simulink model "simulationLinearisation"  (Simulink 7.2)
settings: Solver=ode23  StartTime=0.0  StopTime=2  RelTol=1e-3
undefined symbols (not defined in the file or in its folder): u_b, x_b

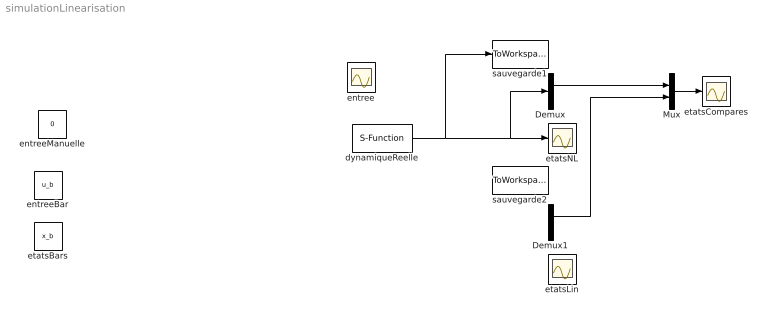
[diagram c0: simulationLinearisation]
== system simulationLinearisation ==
  Demux : Demux  Outputs=2
  Demux1 : Demux  Outputs=2
  Mux : Mux  Inputs=2
  dynamiqueReelle : S-Function  FunctionName=systemeNL  EnableBusSupport=off
  entree : Scope
  entreeBar : Constant  Value=u_b  OutDataType=sfix(16)  OutScaling=2^0
  entreeManuelle : Constant  Value=0  OutDataType=sfix(16)  OutScaling=2^0
  etatsBars : Constant  Value=x_b  OutDataType=sfix(16)  OutScaling=2^0
  etatsCompares : Scope
  etatsLin : Scope
  etatsNL : Scope
  sauvegarde1 : ToWorkspace  VariableName=etatsNL  SampleTime=-1  SaveFormat=Structure With Time
  sauvegarde2 : ToWorkspace  VariableName=etatsLin  SampleTime=-1  SaveFormat=Structure With Time
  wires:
  dynamiqueReelle/1 -> etatsNL/1, Demux/1, sauvegarde1/1
  Demux/1 -> Mux/1
  Demux1/1 -> Mux/2
  Mux/1 -> etatsCompares/1
